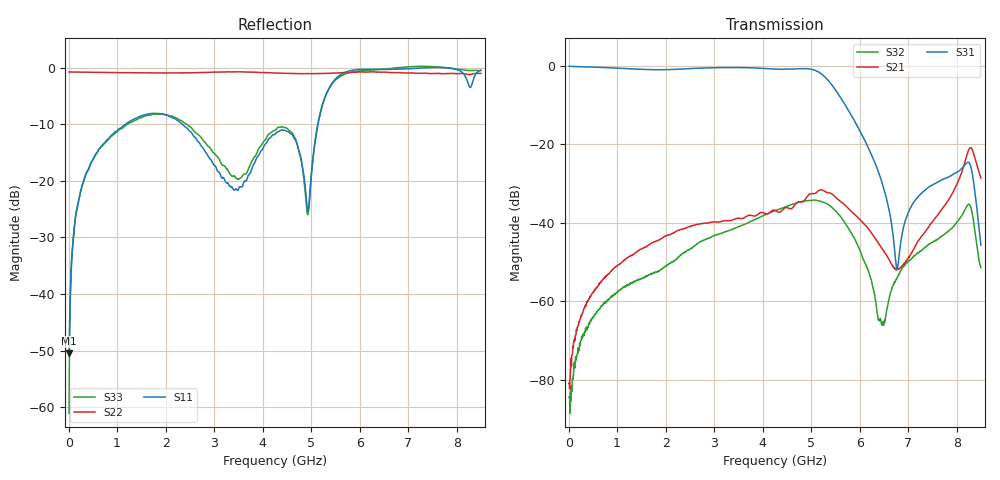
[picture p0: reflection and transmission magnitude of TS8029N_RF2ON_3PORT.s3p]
!Created with skrf (http://scikit-rf.org).
# GHz S RI R 50.0
!freq ReS11 ImS11 ReS12 ImS12 ReS13 ImS13
! ReS21 ImS21 ReS22 ImS22 ReS23 ImS23
! ReS31 ImS31 ReS32 ImS32 ReS33 ImS33
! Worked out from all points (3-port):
!   1601 points, 10 MHz to 8.5 GHz, reference 50 ohm
!   strongest paths, dB at 10 MHz, 2.132 GHz, 4.255 GHz, 6.378 GHz, 8.5 GHz:
!     S31: 0.0, -0.9, -0.8, -26.6, -45.6
!     S21: -80.9, -42.7, -36.8, -44.9, -28.6
!     S32: -84.4, -50.0, -36.8, -64.3, -51.4
!   lowest |S11| = -50.5 dB at 10 MHz (marker M1), VSWR 1.01, Z = 50.3 - j0.0987 ohm
!   |S11| at or under -10 dB: start of sweep to 1.175 GHz; 2.345 GHz to 5.142 GHz (2.796 GHz wide, 74.7 % of centre)
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0.01  0.00284 -0.000981  5.32e-06 3.79e-05  0.9947 -0.00935
      4.46e-05 7.85e-05  -0.9141 0.00479  3.83e-05 1.45e-05
      0.9948 -0.00955  1.58e-05 5.81e-05  0.000569 -0.000678
0.1479625  0.00153 -0.0496  7.25e-05 0.000379  0.9802 -0.0831
           5.4e-05 0.000373  -0.9129 0.0418  4.93e-05 -0.000201
           0.9802 -0.083  3.29e-05 -0.000194  0.000449 -0.0504
0.6626688  -0.0691 -0.1864  -0.000115 0.00176  0.8986 -0.3359
           -0.000112 0.00177  -0.8896 0.1804  -0.000553 -0.000651
           0.8988 -0.3363  -0.000558 -0.000637  -0.0624 -0.1885
4.255  0.23 -0.1168  0.0102 0.0103  -0.7361 -0.5445
       0.0102 0.0103  -0.3367 0.8313  -0.000471 0.0143
       -0.7364 -0.5443  -0.000468 0.0144  0.0408 -0.2774
4.928894  0.0542 -0.00707  0.0179 0.013  -0.9135 0.1388
          0.0179 0.013  -0.1218 0.8754  0.0141 0.013
          -0.9127 0.139  0.0142 0.013  0.0429 -0.0262
5.629319  0.8686 0.1225  0.0159 -0.00924  -0.018 0.3785
          0.0159 -0.00927  0.0372 0.8997  0.00956 -0.00653
          -0.018 0.3785  0.0095 -0.00652  0.8148 -0.2376
6.435869  0.8501 -0.4525  0.00388 -0.00314  0.0215 0.0297
          0.00385 -0.00316  0.1967 0.8879  0.000549 -8.03e-06
          0.0215 0.0298  0.000575 -1.87e-05  0.5197 -0.8144
6.770162  0.8237 -0.5058  0.00252 0.000478  -0.00175 0.00189
          0.00249 0.000473  0.3105 0.8472  0.00012 0.00195
          -0.00177 0.00187  9.57e-05 0.00196  0.4676 -0.8818
8.224075  0.4551 -0.595  0.0707 0.0326  -0.0583 0.00959
          0.0706 0.0326  0.5356 0.689  0.0147 0.00825
          -0.058 0.00948  0.0146 0.00831  0.4 -0.8555
8.5  0.7265 -0.61  0.0114 -0.0355  -0.00248 0.00458
     0.0114 -0.0355  0.6051 0.6497  0.00275 0.000494
     -0.00253 0.00458  0.00266 0.000488  0.3166 -0.8881
